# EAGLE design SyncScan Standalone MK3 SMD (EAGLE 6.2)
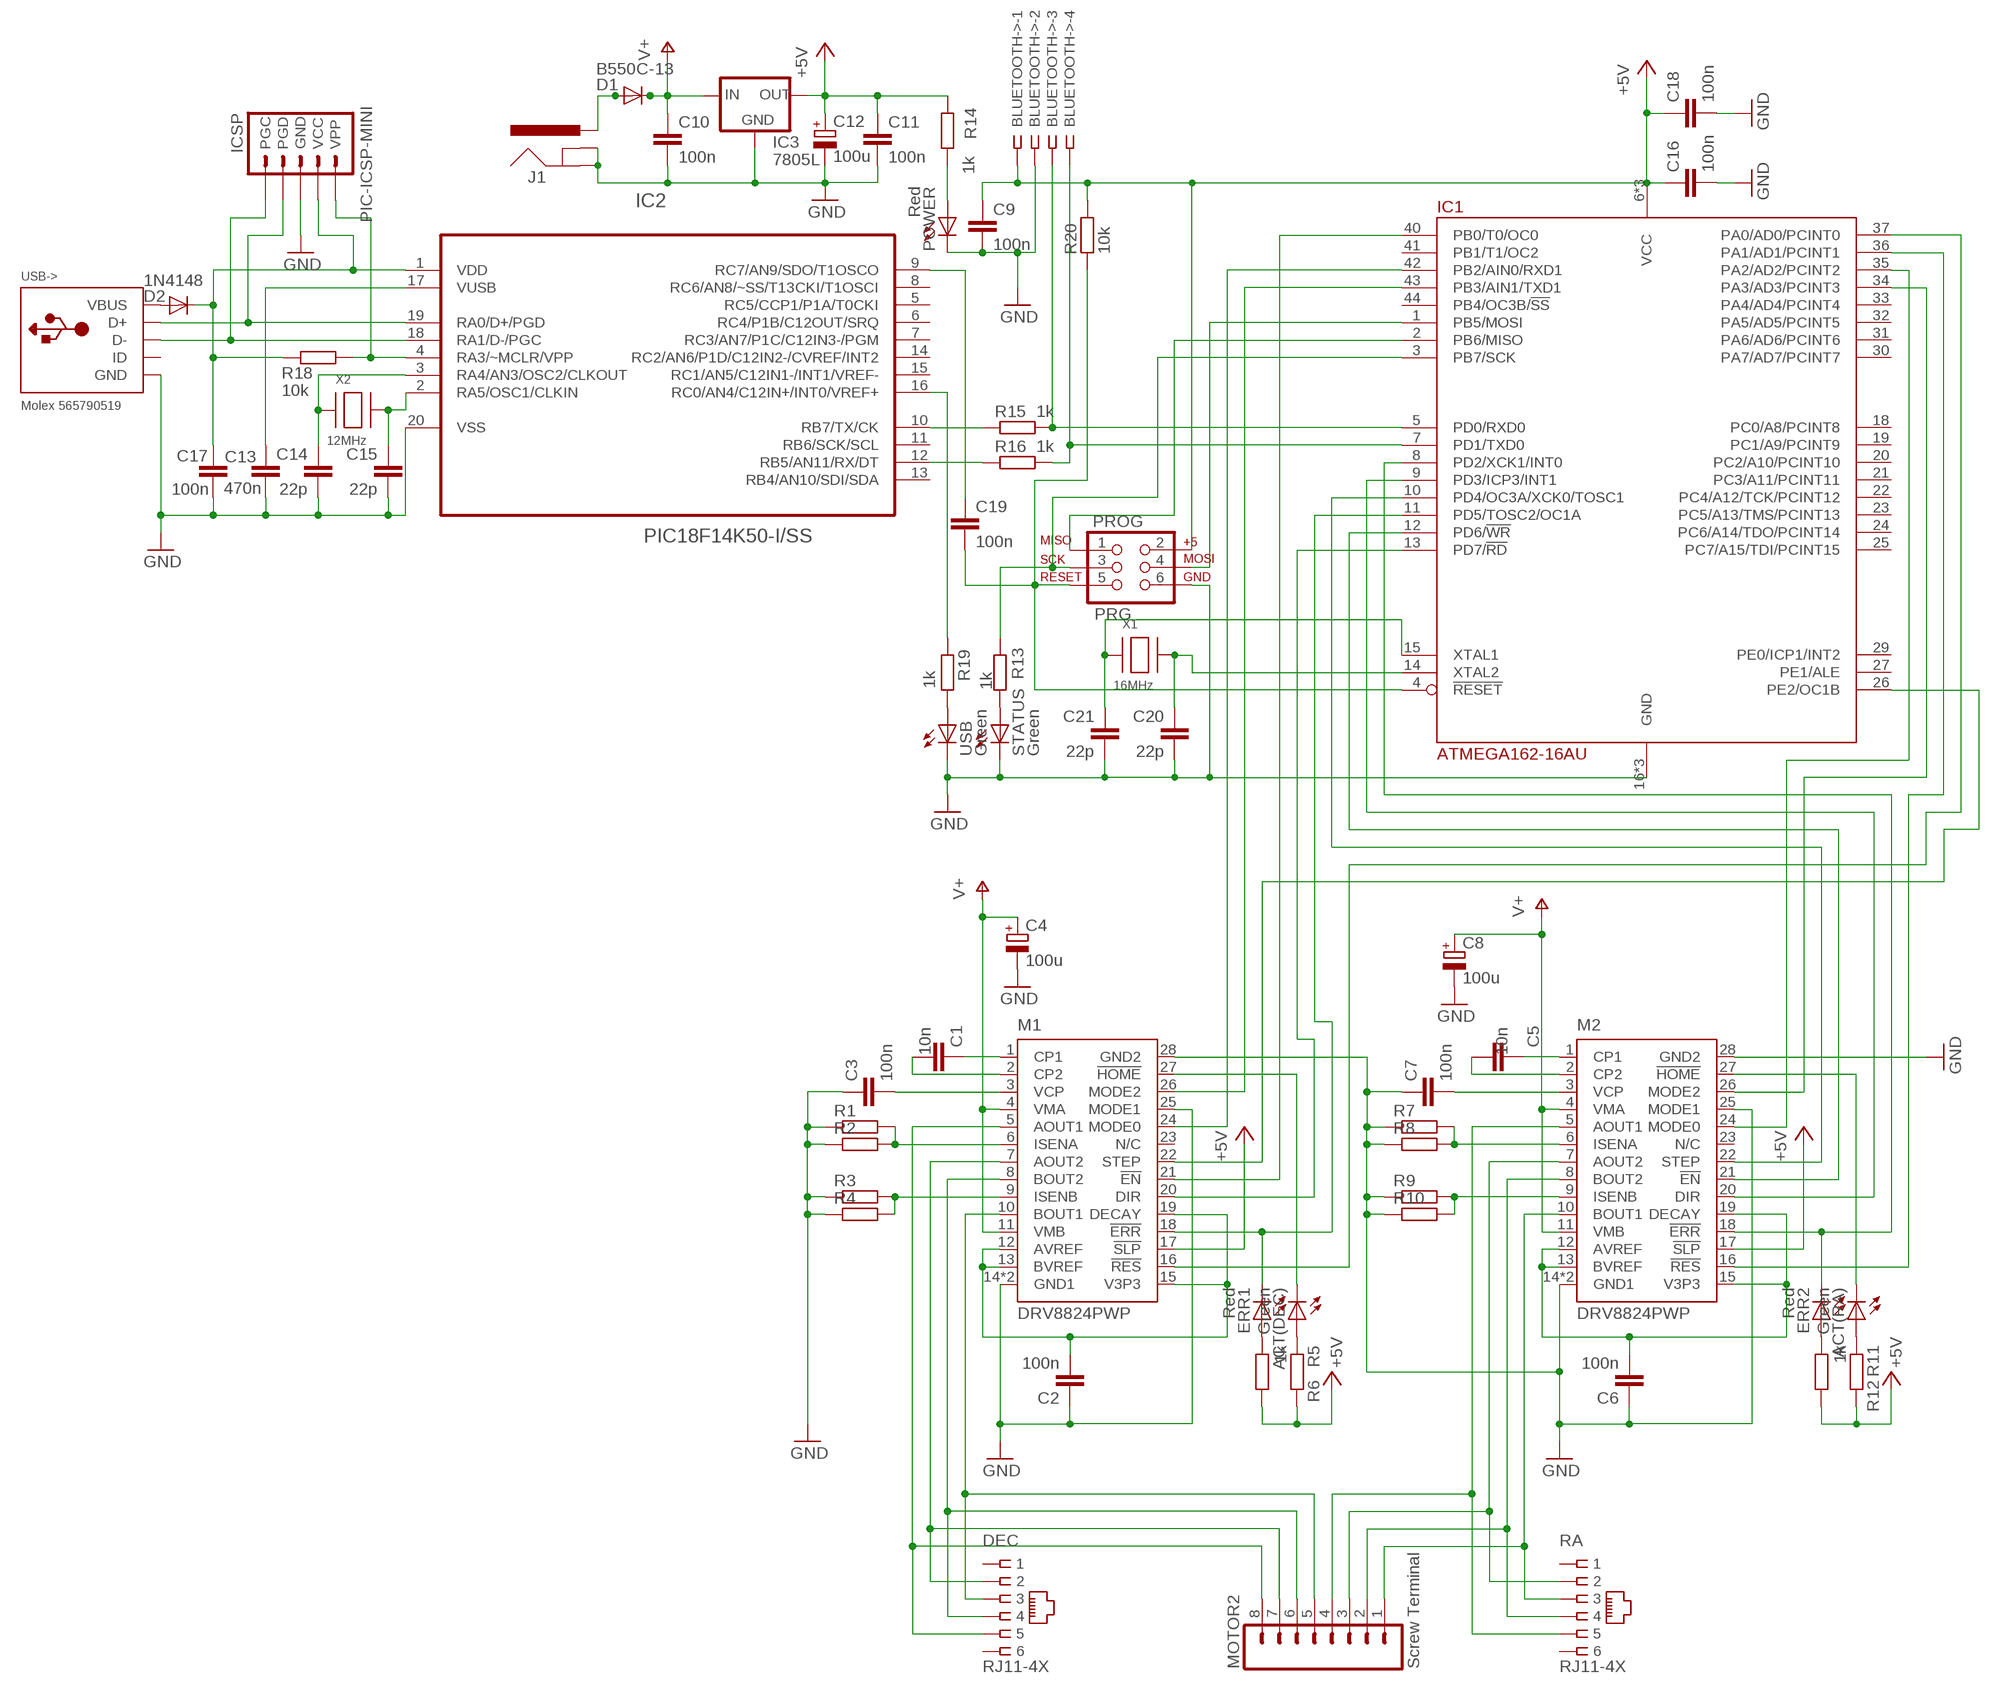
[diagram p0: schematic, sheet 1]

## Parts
ACT(DEC)  Green  LEDSMT1206  [1206]
ACT(RA)  Green  LEDSMT1206  [1206]
BLUETOOTH->  http://www.ebay.co.uk/itm/250991624201  SSW-104-02-S-S-RA  [SSW-104-02-S-S-RA]
C1  10n  C-EUC0603K  [C0603K]
C2  100n  C-EUC0603K  [C0603K]
C3  100n  C-EUC0603K  [C0603K]
C4  100u  CPOL-EUE2.5-6  [E2,5-6]
C5  10n  C-EUC0603K  [C0603K]
C6  100n  C-EUC0603K  [C0603K]
C7  100n  C-EUC0603K  [C0603K]
C8  100u  CPOL-EUE2.5-6  [E2,5-6]
C9  100n  C-EUC0603K  [C0603K]
C10  100n  C-EUC0603K  [C0603K]
C11  100n  C-EUC0603K  [C0603K]
C12  100u  CPOL-EUE2.5-6  [E2,5-6]
C13  470n  C-EUC0603K  [C0603K]
C14  22p  C-EUC0603K  [C0603K]
C15  22p  C-EUC0603K  [C0603K]
C16  100n  C-EUC0603K  [C0603K]
C17  100n  C-EUC0603K  [C0603K]
C18  100n  C-EUC0603K  [C0603K]
C19  100n  C-EUC0603K  [C0603K]
C20  22p  C-EUC0603K  [C0603K]
C21  22p  C-EUC0603K  [C0603K]
D1  B550C-13  DIODE-SMC  [SMC]
D2  1N4148  DIODESOD  [SOD-323]
DEC  RJ11-4X  [RJ11-NO_SHIELD]
ERR1  Red  LEDSMT1206  [1206]
ERR2  Red  LEDSMT1206  [1206]
IC1  ATMEGA162-16AU  [TQFP44]
IC2  PIC18F14K50-I/SS  [SSOP20]
IC3  7805L  78LXXSOT-23  [SOT23]
ICSP  PIC-ICSP-MINI  [PIC-ICSP-MINI]
J1  POWER_JACKSMD  [POWER_JACK_SMD]
M1  DRV8824PWP  [HTSSOP28PWP]
M2  DRV8824PWP  [HTSSOP28PWP]
MOTOR2  Screw Terminal  M083.5MM-8  [SCREWTERMINAL-3.5MM-8]
POWER  Red  LEDSMT1206  [1206]
PROG  PRG  AVR_SPI_PRG_6PTH  [2X3]
R1  1.5R  R-EU_R2512  [R2512]
R2  1.5R  R-EU_R2512  [R2512]
R3  1.5R  R-EU_R2512  [R2512]
R4  1.5R  R-EU_R2512  [R2512]
R5  1k  R-EU_R0603  [R0603]
R6  1k  R-EU_R0603  [R0603]
R7  1.5R  R-EU_R2512  [R2512]
R8  1.5R  R-EU_R2512  [R2512]
R9  1.5R  R-EU_R2512  [R2512]
R10  1.5R  R-EU_R2512  [R2512]
R11  1k  R-EU_R0603  [R0603]
R12  1k  R-EU_R0603  [R0603]
R13  1k  R-EU_R0603  [R0603]
R14  1k  R-EU_R0603  [R0603]
R15  1k  R-EU_R0603  [R0603]
R16  1k  R-EU_R0603  [R0603]
R18  10k  R-EU_R0603  [R0603]
R19  1k  R-EU_R0603  [R0603]
R20  10k  R-EU_R0603  [R0603]
RA  RJ11-4X  [RJ11-NO_SHIELD]
STATUS  Green  LEDSMT1206  [1206]
USB  Green  LEDSMT1206  [1206]
USB->  Molex 565790519  USBMOLEX  [USB-MINIB-THM-MOLEX]
X1  16MHz  XTALNX5032  [NX5032]
X2  12MHz  XTALNX5032  [NX5032]

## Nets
3.3V-1: C2.2 M1.12(AVREF) M1.13(BVREF) M1.15(V3P3) M1.19(DECAY)
3.3V-2: C6.2 M2.12(AVREF) M2.13(BVREF) M2.15(V3P3) M2.19(DECAY)
!EN-1: IC1.40(PB0/T0/OC0) M1.21(!EN)
!EN-2: IC1.12(PD6/!WR) M2.21(!EN)
!ERR-1: ERR1.C IC1.11(PD5/TOSC2/OC1A) M1.18(!ERR)
!ERR-2: ERR2.C IC1.8(PD2/XCK1/INT0) M2.18(!ERR)
!HOME-1: ACT(DEC).C M1.27(!HOME)
!HOME-2: ACT(RA).C M2.27(!HOME)
!RST-1: IC1.37(PA0/AD0/PCINT0) M1.16(!RES)
!RST-2: IC1.36(PA1/AD1/PCINT1) M2.16(!RES)
+5V: BLUETOOTH->.1 C9.1 C11.1 C12.+ C16.1 C18.1 IC1.6(VCC) IC1.17(VCC) IC1.38(VCC) IC3.1(OUT) M1.17(!SLP) M2.17(!SLP) PROG.2 R5.2 R6.2 R11.2 R12.2 R14.1 R20.2
A1-1: DEC.5 M1.5(AOUT1) MOTOR2.8
A1-2: M2.5(AOUT1) MOTOR2.4 RA.5
A2-1: DEC.2 M1.7(AOUT2) MOTOR2.7
A2-2: M2.7(AOUT2) MOTOR2.3 RA.2
AVROSC1: C21.1 IC1.15(XTAL1) X1.P$1
AVROSC2: C20.1 IC1.14(XTAL2) X1.P$2
B1-1: DEC.3 M1.10(BOUT1) MOTOR2.5
B1-2: M2.10(BOUT1) MOTOR2.1 RA.3
B2-1: DEC.4 M1.8(BOUT2) MOTOR2.6
B2-2: M2.8(BOUT2) MOTOR2.2 RA.4
CP1-1: C1.1 M1.1(CP1)
CP1-2: C5.1 M2.1(CP1)
CP2-1: C1.2 M1.2(CP2)
CP2-2: C5.2 M2.2(CP2)
D+: IC2.19(RA0/D+/PGD) ICSP.4(PGD) USB->.D+
D-: IC2.18(RA1/D-/PGC) ICSP.5(PGC) USB->.D-
DIR-1: IC1.13(PD7/!RD) M1.20(DIR)
DIR-2: IC1.9(PD3/ICP3/INT1) M2.20(DIR)
GND: BLUETOOTH->.2 C2.1 C3.1 C4.- C6.1 C7.1 C8.- C9.2 C10.2 C11.2 C12.- C13.1 C14.2 C15.2 C16.2 C17.2 C18.2 C20.2 C21.2 IC1.16(GND) IC1.28(GND) IC1.39(GND) IC2.20(VSS) IC3.3(GND) ICSP.3(GND) J1.GND(GNDBREAK) J1.P$4(GND) M1.14(GND1) M1.25(MODE1) M1.28(GND2) M1.EXP(GND1) M2.14(GND1) M2.25(MODE1) M2.28(GND2) M2.EXP(GND1) POWER.C PROG.6 R1.1 R2.1 R3.1 R4.1 R7.1 R8.1 R9.1 R10.1 STATUS.C USB->.GND USB.C
ISENA-1: M1.6(ISENA) R1.2 R2.2
ISENA-2: M2.6(ISENA) R7.2 R8.2
ISENB-1: M1.9(ISENB) R3.2 R4.2
ISENB-2: M2.9(ISENB) R9.2 R10.2
LED1: ERR1.A R6.1
LED2: ACT(DEC).A R5.1
LED3: ERR2.A R12.1
LED4: ACT(RA).A R11.1
M0-1: IC1.42(PB2/AIN0/RXD1) M1.24(MODE0)
M0-2: IC1.35(PA2/AD2/PCINT2) M2.24(MODE0)
M2-1: IC1.43(PB3/AIN1/TXD1) M1.26(MODE2)
M2-2: IC1.34(PA3/AD3/PCINT3) M2.26(MODE2)
MCLR: IC2.4(RA3/~MCLR/VPP) ICSP.1(VPP) R18.1
MISO: IC1.2(PB6/MISO) PROG.1
MOSI: IC1.1(PB5/MOSI) PROG.4
N$1: C3.2 M1.3(VCP)
N$2: C19.1 IC2.9(RC7/AN9/SDO/T1OSCO)
PWRLED: POWER.A R14.2
RESET: C19.2 IC1.4(!RESET) PROG.5 R20.1
RX(BTH): BLUETOOTH->.4 IC1.7(PD1/TXD0) R16.1
RX(USB): IC2.12(RB5/AN11/RX/DT) R16.2
SCLK: IC1.3(PB7/SCK) PROG.3 R13.1
STATLED: R13.2 STATUS.A
STEP-1: IC1.26(PE2/OC1B) M1.22(STEP)
STEP-2: IC1.10(PD4/OC3A/XCK0/TOSC1) M2.22(STEP)
TX(BTH): BLUETOOTH->.3 IC1.5(PD0/RXD0) R15.1
TX(USB): IC2.10(RB7/TX/CK) R15.2
USBLED: R19.1 USB.A
USBOSC1: C15.1 IC2.2(RA5/OSC1/CLKIN) X2.P$2
USBOSC2: C14.1 IC2.3(RA4/AN3/OSC2/CLKOUT) X2.P$1
USBSTAT: IC2.16(RC0/AN4/C12IN+/INT0/VREF+) R19.2
V+: C4.+ C8.+ C10.1 D1.C IC3.2(IN) M1.4(VMA) M1.11(VMB) M2.4(VMA) M2.11(VMB)
VBUS: D2.2(A) USB->.VBUS
VCP-2: C7.2 M2.3(VCP)
VIN: D1.A J1.VIN0(PWR) J1.VIN1(PWR)
VPIC: C17.1 D2.1(C) IC2.1(VDD) ICSP.2(VCC) R18.2
VUSB: C13.2 IC2.17(VUSB)
Unconnected: DEC.1 DEC.6 IC1.18(PC0/A8/PCINT8) IC1.19(PC1/A9/PCINT9) IC1.20(PC2/A10/PCINT10) IC1.21(PC3/A11/PCINT11) IC1.22(PC4/A12/TCK/PCINT12) IC1.23(PC5/A13/TMS/PCINT13) IC1.24(PC6/A14/TDO/PCINT14) IC1.25(PC7/A15/TDI/PCINT15) IC1.27(PE1/ALE) IC1.29(PE0/ICP1/INT2) IC1.30(PA7/AD7/PCINT7) IC1.31(PA6/AD6/PCINT6) IC1.32(PA5/AD5/PCINT5) IC1.33(PA4/AD4/PCINT4) IC1.41(PB1/T1/OC2) IC1.44(PB4/OC3B/!SS) IC2.5(RC5/CCP1/P1A/T0CKI) IC2.6(RC4/P1B/C12OUT/SRQ) IC2.7(RC3/AN7/P1C/C12IN3-/PGM) IC2.8(RC6/AN8/~SS/T13CKI/T1OSCI) IC2.11(RB6/SCK/SCL) IC2.13(RB4/AN10/SDI/SDA) IC2.14(RC2/AN6/P1D/C12IN2-/CVREF/INT2) IC2.15(RC1/AN5/C12IN1-/INT1/VREF-) M1.23(N/C) M2.23(N/C) RA.1 RA.6 USB->.ID

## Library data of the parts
ACT(DEC) ACT(RA) STATUS USB = led:LED: LED; MF: KINGBRIGHT; MPN: L-424GDT; OC_FARNELL: 1142496
BLUETOOTH-> = con-samtec:SSW-104-02-S-S: THROUGH-HOLE .025" SQ POST SOCKET Source: Samtec SSW.pdf; OC_FARNELL: unknown; OC_NEWARK: 11P9385
C1 C5 = resistor:C-EU: CAPACITOR, European symbol; MF: KEMET; MPN: C0603C103K1RACTU; OC_FARNELL: 1865545
C2 C3 C6 C7 C9-C11 C16-C19 = resistor:C-EU: CAPACITOR, European symbol; MF: KEMET; MPN: C0603C104K4RACTU; OC_FARNELL: 1414610
C4 C8 C12 = resistor:CPOL-EU: POLARIZED CAPACITOR, European symbol; MF: MULTICOMP; MPN: MCGPR25V107M6.3X11; OC_FARNELL: 9451188
C13 = rcl:C-EU: CAPACITOR, European symbol; MF: AVX; MPN: 0603ZD474KAT2A; OC_FARNELL: 1833805
C14 C15 C20 C21 = rcl:C-EU: CAPACITOR, European symbol; MF: MULTICOMP; MPN: U0603C220JCT; OC_FARNELL: 9406107
D1 = diode:DIODE-: DIODE; MF: DIODES INC.; MPN: B550C-13-F; OC_FARNELL: 1858608
D2 = SparkFun:DIODE: Diode; MF: MULTICOMP; MPN: 1N4148.; OC_FARNELL: 9565124
DEC RA = con-tycoelectronics:RJ11: CORCOM Modular RJ Jacks No Shield Source: www.tycoelectronics.com .. ENG_DS_1654001_1099_RJ_L_0507.pdf; MF: MH CONNECTORS; MPN: MHRJJ64NFRA; OC_FARNELL: 3938347; OC_NEWARK: 19R7022
ERR1 ERR2 POWER = led:LED: LED; MF: KINGBRIGHT; MPN: L-424HDT; OC_FARNELL: 1142499
IC1 = atmel:ATMEGA162: 8-bit RISC MICROCONTROLLER 16K Bytes internal flash program memory 1K Bytes internal SRAM Upto 64K Bytes optional external memory space 512 Bytes EEPROM Two 8-bit timers Two 16-bit timers Dual programmable serial USARTs Master/Slave serial SPI interface Source: ATMEGA162_DIP40.lbr; MF: ATMEL; MPN: ATMEGA162-16AU; OC_FARNELL: 9171150
IC2 = microchip:PIC18F14K50: USB Flash Microcontrollers; MF: MICROCHIP; MPN: PIC18F14K50-I/SS; OC_FARNELL: 1648504
IC3 = v-reg:78LXX: VOLTAGE REGULATOR; MF: TAIWAN SEMICONDUCTOR; MPN: TS78L05CX RF; OC_FARNELL: 1476698
ICSP = SparkFun:PIC-ICSP-MINI: PIC-ICSP-Mini Miniature 5-pin connection for temporary programming of PICs. Use this device in your design to save space. Program the PIC with this adapter Spark Fun Electronics SKU : BOB-00194; OC_FARNELL: unknown
J1 = SparkFun:POWER_JACK: Power Jack This is the standard 5.5mm barrel jack for power. The PTH is the most common, proven, reliable, footprint. All others are experimental. The Slot footprint only works if the mill layer is transmitted to the PCB fab house so be warned. Spark Fun Electronics SKU : PRT-00119. Mating wall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; MF: MULTICOMP; MPN: MJ-179SMT; OC_FARNELL: 1737262
M1 M2 = texas:DRV8824; MF: TEXAS INSTRUMENTS; MPN: DRV8824PWP; OC_FARNELL: 1815786
MOTOR2 = SparkFun:M08: Header 8 Standard 8-pin 0.1" header. Use with straight break away headers (SKU : PRT-00116), right angle break away headers (PRT-00553), swiss pins (PRT-00743), machine pins (PRT-00117), and female headers (PRT-00115).; MF: LUMBERG; MPN: KRMC 08; OC_FARNELL: 1217307
PROG = SparkFun:AVR_SPI_PRG_6: AVR ISP 6 Pin This is the reduced ISP connector for AVR programming. Common on Arduino. This footprint will take up less PCB space and can be used with a 10-pin to 6-pin adapter such as SKU: BOB-08508; MF: TE CONNECTIVITY / AMP; MPN: 826632-3; OC_FARNELL: 3418492
R1-R4 R7-R10 = resistor:R-EU_: RESISTOR, European symbol; MF: YAGEO (PHYCOMP); MPN: RC2512FK-7W1R5L; OC_FARNELL: 1840520
R5 R6 R11 R12 = resistor:R-EU_: RESISTOR, European symbol; MF: VISHAY DRALORIC; MPN: CRCW06031K00FKEA; OC_FARNELL: 1469740
R13 R14 R19 = rcl:R-EU_: RESISTOR, European symbol; MF: VISHAY DRALORIC; MPN: CRCW06031K00FKEA; OC_FARNELL: 1469740
R15 R16 = SmartPrj:R-EU_: RESISTOR, European symbol; MF: VISHAY DRALORIC; MPN: CRCW06031K00FKEA; OC_FARNELL: 1469740
R18 R20 = rcl:R-EU_: RESISTOR, European symbol; MF: VISHAY DRALORIC; MPN: CRCW060310K0FKEA; OC_FARNELL: 1469748
USB-> = adafruit:USB: USB Connectors USBMINIB - Surface Mount Female Mini-B USB Connector 4UConnector: 06564 By microbuilder.eu Thru-hole RA Female Mini-B USB Connector 4UConnector: 18732 By ladyada.net; MF: MOLEX; MPN: 565790519; OC_FARNELL: 1125347
X1 = adafruit:XTAL: Low cost SMT crystals, no capacitors included; MF: TXC; MPN: 7A-16.000MAAJ-T; OC_FARNELL: 1841946
X2 = adafruit:XTAL: Low cost SMT crystals, no capacitors included; MF: TXC; MPN: 7A-12.000MAAJ-T; OC_FARNELL: 1841940

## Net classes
1 power: width 0.61 mm, drill 0.711 mm, clearance 0.203 mm
2 gnd: width 0.305 mm, drill 0.711 mm, clearance 0.203 mm
3 usbvcc: width 0.508 mm, drill 0.711 mm, clearance 0.203 mm

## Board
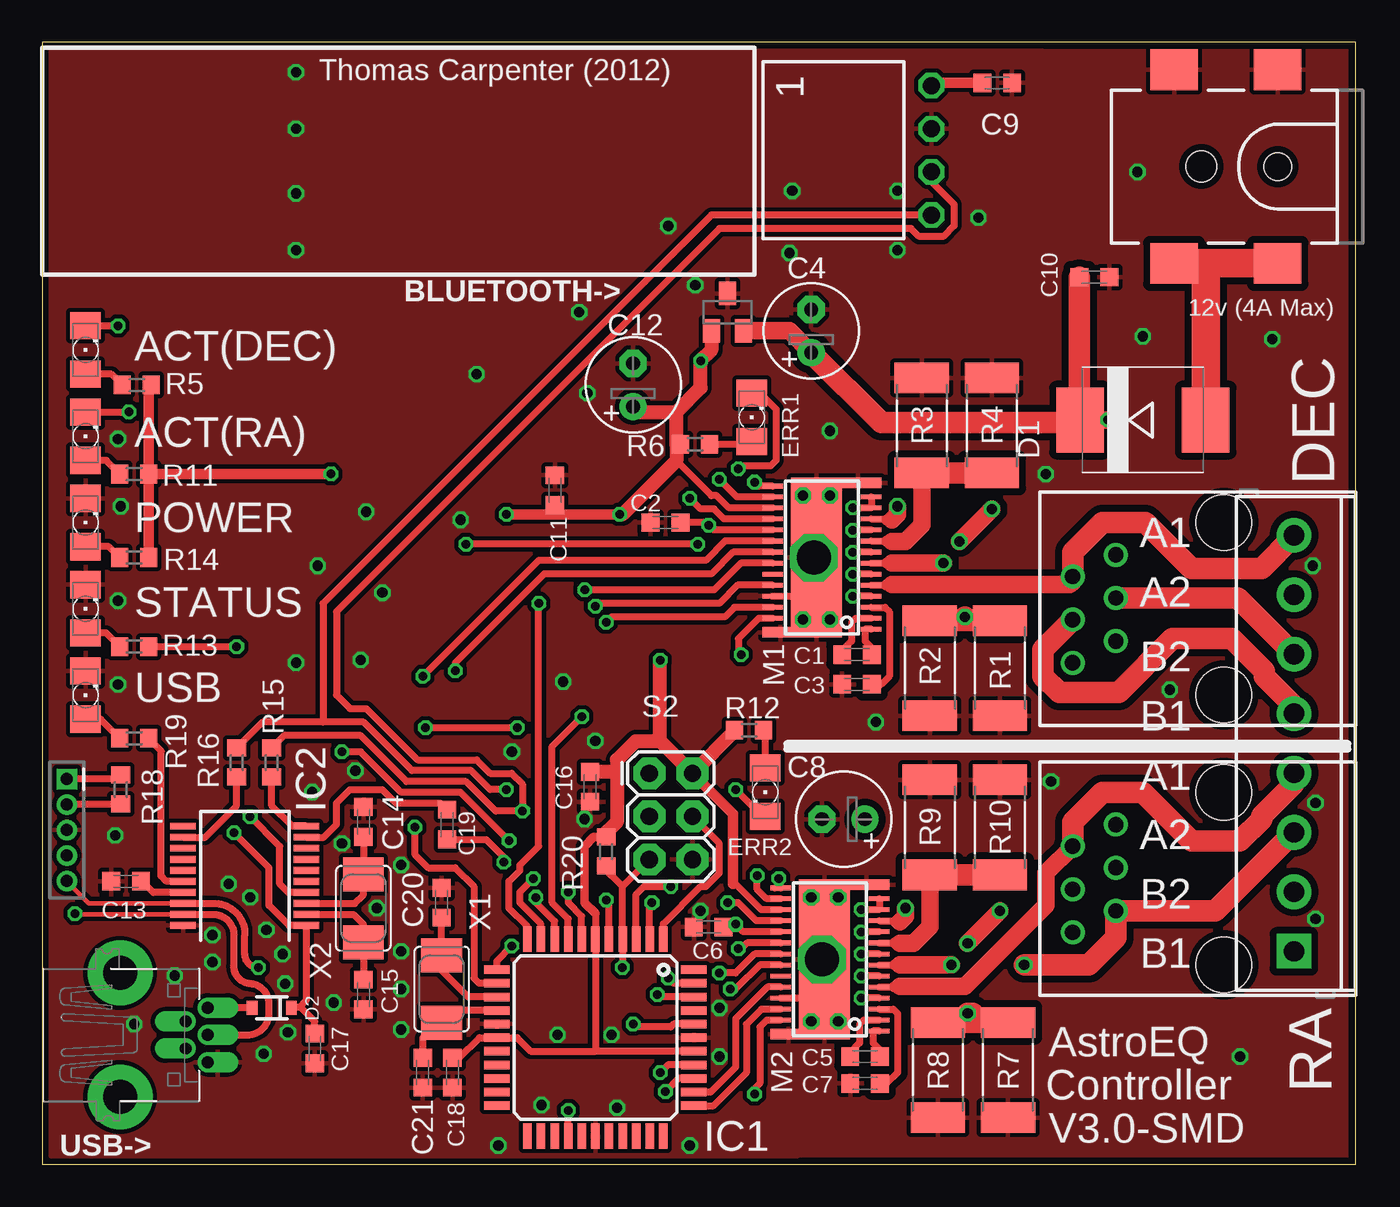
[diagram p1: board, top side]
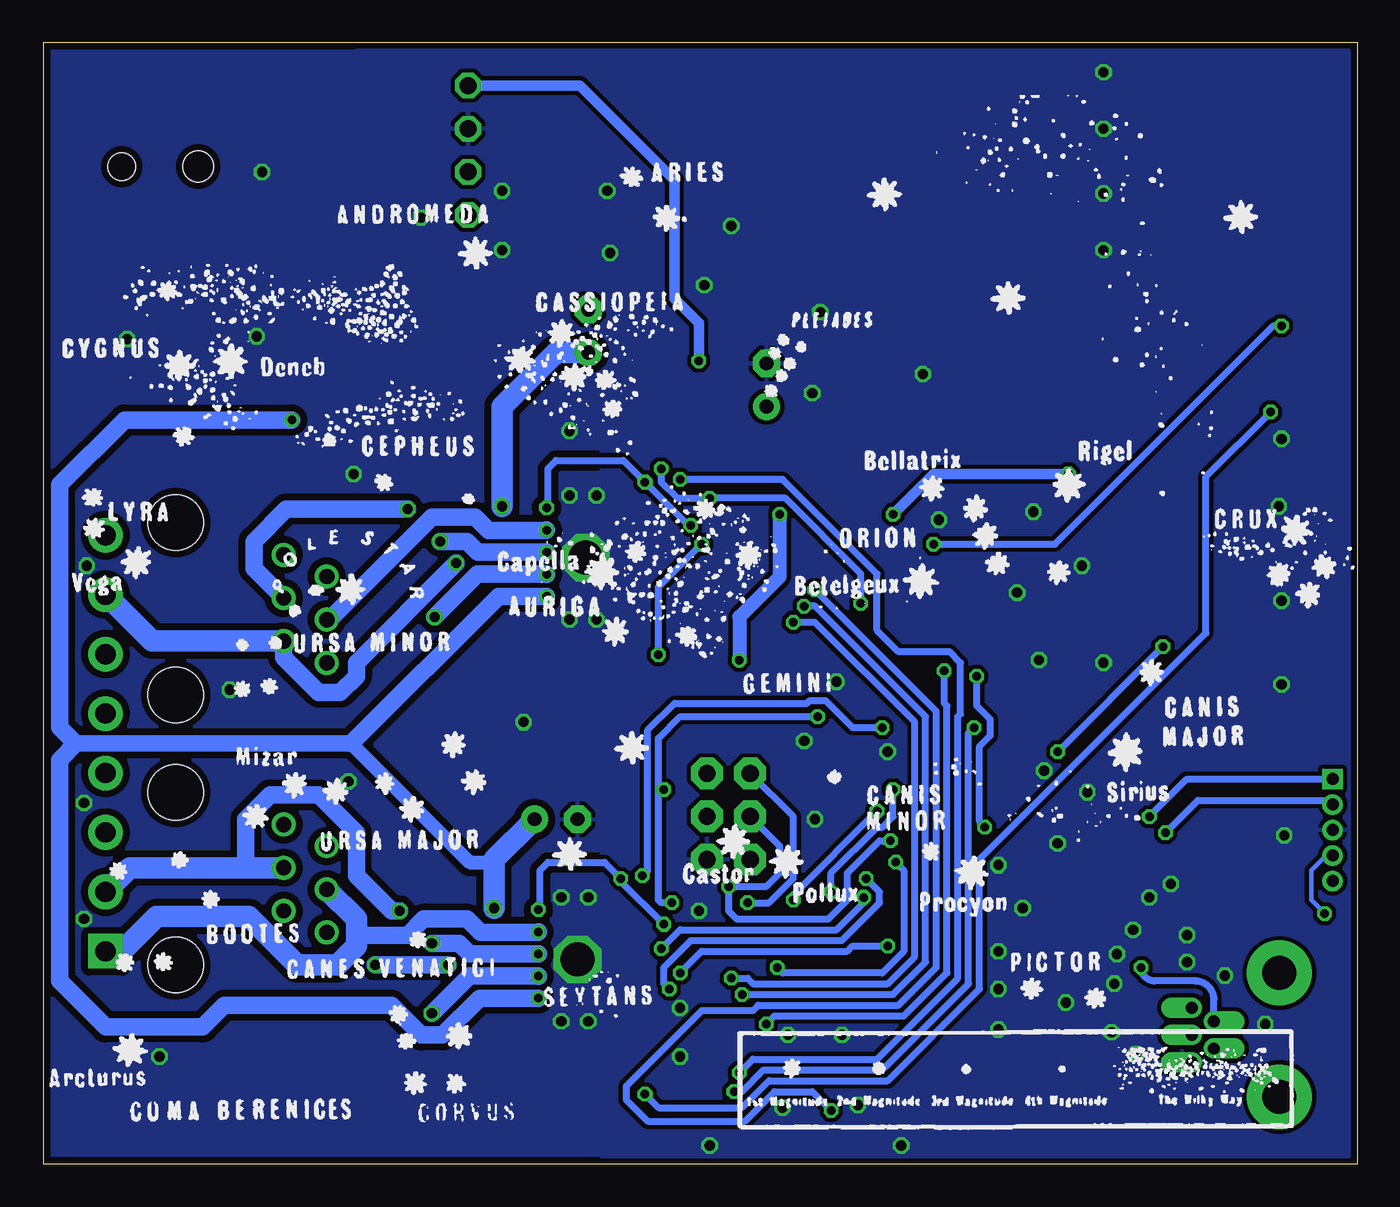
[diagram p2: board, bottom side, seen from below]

Size 77.31 x 66.04 mm. Coordinates in mm from the lower left corner, seen from the top.
Outline: 0,66.04 0,0 77.31,0 77.31,66.04 0,66.04
Copper layers (1*16): Top 0.035mm / dielectric 1.5mm / Bottom 0.035mm
Design rules: minimum track width 0.2mm, minimum drill 0.5mm, track to track 0.2mm, track to pad 0.2mm, pad to pad 0.2mm, via to via 0.2mm, smd to smd 0mil, copper to edge 10mil, drill to drill 0.2mm, minimum pad ring 10mil, minimum via ring 7mil, stop-mask expansion 0.125mm, vias tented up to drill 0mil, thermal gap 10mil

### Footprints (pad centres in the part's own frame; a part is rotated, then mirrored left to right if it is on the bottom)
1206 = smd 1.6 x 1.803: A -1.422,0; C 1.422,0
SSW-104-02-S-S-RA = drill 1 pad 1.5 octagon: 1 -3.81,1.524; 2 -1.27,1.524; 3 1.27,1.524; 4 3.81,1.524
C0603K = smd 1.05 x 1.08: 1 -0.875,0; 2 0.875,0
E2,5-6 = drill 0.813 pad 1.6: + -1.27,0 | drill 0.813 pad 1.6 octagon: - 1.27,0
SMC = smd 2.8 x 3.8: A 3.7,0; C -3.7,0
SOD-323 = smd 0.63 x 0.83: 1 -1.15,0; 2 1.15,0
RJ11-NO_SHIELD = drill 0.9 pad 1.4: 1 -3.175,8.89; 2 -1.905,6.35; 3 -0.635,8.89; 4 0.635,6.35; 5 1.905,8.89; 6 3.175,6.35 | hole 3.251: -5.08,0; 5.08,0
TQFP44 = smd 1.5 x 0.5: 1 -5.8,4; 2 -5.8,3.2; 3 -5.8,2.4; 4 -5.8,1.6; 5 -5.8,0.8; 6 -5.8,0; 7 -5.8,-0.8; 8 -5.8,-1.6; 9 -5.8,-2.4; 10 -5.8,-3.2; 11 -5.8,-4; 23 5.8,-4; 24 5.8,-3.2; 25 5.8,-2.4; 26 5.8,-1.6; 27 5.8,-0.8; 28 5.8,0; 29 5.8,0.8; 30 5.8,1.6; 31 5.8,2.4; 32 5.8,3.2; 33 5.8,4 | smd 0.5 x 1.5: 12 -4,-5.8; 13 -3.2,-5.8; 14 -2.4,-5.8; 15 -1.6,-5.8; 16 -0.8,-5.8; 17 0,-5.8; 18 0.8,-5.8; 19 1.6,-5.8; 20 2.4,-5.8; 21 3.2,-5.8; 22 4,-5.8; 34 4,5.8; 35 3.2,5.8; 36 2.4,5.8; 37 1.6,5.8; 38 0.8,5.8; 39 0,5.8; 40 -0.8,5.8; 41 -1.6,5.8; 42 -2.4,5.8; 43 -3.2,5.8; 44 -4,5.8
SSOP20 = smd 0.4 x 1.5: 1 -2.925,-3.625; 2 -2.275,-3.625; 3 -1.625,-3.625; 4 -0.975,-3.625; 5 -0.325,-3.625; 6 0.325,-3.625; 7 0.975,-3.625; 8 1.625,-3.625; 9 2.275,-3.625; 10 2.925,-3.625; 11 2.925,3.625; 12 2.275,3.625; 13 1.625,3.625; 14 0.975,3.625; 15 0.325,3.625; 16 -0.325,3.625; 17 -0.975,3.625; 18 -1.625,3.625; 19 -2.275,3.625; 20 -2.925,3.625
SOT23 = smd 1 x 1.4: 1 -0.95,-1.1; 2 0.95,-1.1; 3 0,1.1
PIC-ICSP-MINI = drill 0.7 square: 1 -3,0 | drill 0.7: 2 -1.5,0; 3 0,0; 4 1.5,0; 5 3,0
POWER_JACK_SMD = smd 2.8 x 2.4: GND 0,-5.7; P$4 6.1,-5.7; VIN0 0,5.7; VIN1 6.1,5.7 | hole 1.6: 0,0 | hole 1.8: 4.5,0
HTSSOP28PWP = smd 0.27 x 1.2: 1 -4.21,-2.9; 2 -3.575,-2.9; 3 -2.925,-2.9; 4 -2.275,-2.9; 5 -1.625,-2.9; 6 -0.975,-2.9; 7 -0.325,-2.9; 8 0.325,-2.9; 9 0.975,-2.9; 10 1.625,-2.9; 11 2.275,-2.9; 12 2.925,-2.9; 13 3.575,-2.9; 15 4.21,2.9; 16 3.575,2.9; 17 2.925,2.9; 18 2.275,2.9; 19 1.625,2.9; 20 0.975,2.9; 21 0.325,2.9; 22 -0.325,2.9; 23 -0.975,2.9; 24 -1.625,2.9; 25 -2.275,2.9; 26 -2.925,2.9; 27 -3.575,2.9 | smd 0.61 x 2.735: 14 4.395,-2.132 | smd 0.61 x 2.1: 28 -4.395,2.45 | smd 9.4 x 3: EXP 0,0.318
SCREWTERMINAL-3.5MM-8 = drill 1.2 pad 2.032 square: 1 0,0 | drill 1.2 pad 2.032: 2 3.5,0; 3 7,0; 4 10.5,0; 5 14,0; 6 17.5,0; 7 21,0; 8 24.5,0
2X3 = drill 1.016 pad 1.88 octagon: 1 0,0; 2 0,2.54; 3 2.54,0; 4 2.54,2.54; 5 5.08,0; 6 5.08,2.54
R2512 = smd 1.8 x 3.2: 1 -2.8,0; 2 2.8,0
R0603 = smd 1 x 1.1: 1 -0.85,0; 2 0.85,0
USB-MINIB-THM-MOLEX = drill 0.7 offset: D+ 0,9.72; D- -0.8,8.42; GND 1.6,9.72; ID 0.8,8.42; VBUS -1.6,9.72 | drill 2 pad 3.81: GND1 -3.65,4.57; GND4 3.65,4.57
NX5032 = smd 2 x 2.4: P$1 2,0; P$2 -2,0

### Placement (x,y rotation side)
ACT(DEC)  2.54,47.94 90 top
ACT(RA)  2.54,42.86 90 top
BLUETOOTH->  50.8,59.69 270 top
C1  47.94,30 180 top
C2  36.67,37.78 0 top
C3  47.94,28.26 0 top
C4  45.24,49.05 90 top
C5  48.42,6.35 180 top
C6  39.21,13.97 0 top
C7  48.42,4.76 0 top
C8  47.15,20.32 180 top
C9  56.2,63.66 0 top
C10  61.91,52.23 0 top
C11  30.16,39.69 90 top
C12  34.77,45.88 90 top
C13  4.92,16.67 0 top
C14  18.89,20.16 90 top
C15  18.89,10 270 top
C16  32.23,22.23 270 top
C17  16.03,6.83 270 top
C18  24.13,5.4 270 top
C19  23.81,20 270 top
C20  23.5,15.4 90 top
C21  22.38,5.4 270 top
D1  64.77,43.81 0 top
D2  13.49,9.21 180 top
DEC  69.53,32.7 90 top
ERR1  41.75,43.97 90 top
ERR2  42.55,21.91 270 top
IC1  32.54,7.46 270 top
IC2  11.91,16.99 90 top
IC3  40.32,50.16 0 top
ICSP  1.43,19.68 270 top
J1  72.71,58.74 180 top
M1  45.88,35.72 90 top
M2  46.35,12.06 90 top
MOTOR2  73.66,12.54 90 top
POWER  2.54,37.78 90 top
PROG  35.72,23.02 270 top
R1  56.36,29.21 90 top
R2  52.23,29.21 90 top
R3  51.75,43.5 270 top
R4  55.88,43.5 270 top
R5  5.56,45.88 0 top
R6  38.42,42.39 180 top
R7  56.83,5.56 90 top
R8  52.7,5.56 90 top
R9  52.23,19.84 270 top
R10  56.36,19.84 270 top
R11  5.4,40.64 0 top
R12  41.59,25.56 180 top
R13  5.4,30.48 180 top
R14  5.4,35.72 180 top
R15  13.49,23.65 270 top
R16  11.43,23.65 270 top
R18  4.6,22.07 270 top
R19  5.4,25.08 0 top
R20  33.18,18.41 90 top
RA  69.53,16.83 90 top
STATUS  2.54,32.7 90 top
USB  2.54,27.62 90 top
USB->  0,7.62 270 top
X1  23.5,10.32 270 top
X2  18.89,15.08 90 top

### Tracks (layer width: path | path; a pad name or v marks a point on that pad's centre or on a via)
3.3V-1  (via drill 0.5)
  Top 0.406: v47.7,38.66 47.72,38.64 M1.12 M1.13 | M1.15 42.15,39.93 v41.91,40.16 | M1.19 39.49,37.34 v39.21,37.62 39.05,37.78 C2.2
  Bottom 0.406: v47.7,38.66 47.62,38.73 47.62,40.96 47.15,41.43 43.18,41.43 v41.91,40.16 39.37,37.62 v39.21,37.62
3.3V-2  (via drill 0.5)
  Top 0.406: v48.18,15 48.19,14.99 M2.12 M2.13 | 43.1,16.27 M2.15 43.45,16.39 43.34,16.51 v43.34,16.83 | M2.19 41.24,13.69 v40.8,14.13 40.64,13.97 C6.2
  Bottom 0.406: v48.18,15 48.1,15.08 48.1,17.3 47.62,17.78 44.29,17.78 v43.34,16.83 43.34,16.67 v40.8,14.13
!EN-1  (via drill 0.5)
  Top 0.406: M1.21 40.65,36.04 39.37,34.77 29.53,34.77 24.29,29.53 v24.29,29.05 | IC1.40 37.15,8.26 36.99,8.1 34.92,8.1 v34.77,8.26 v34.76,8.26
  Bottom 0.406: v34.77,8.26 34.29,8.73 26.67,8.73 24.13,11.27 24.13,26.99 24.29,27.15 v24.29,29.05
!EN-2  (via drill 0.5)
  Top 0.406: M2.21 41.92,12.39 40.8,11.27 v39.85,11.27 | IC1.12 26.74,11.98 v27.62,12.86
  Bottom 0.406: v39.85,11.27 38.58,12.54 30,12.54 29.69,12.86 v27.62,12.86
!ERR-1  (via drill 0.5)
  Top 0.406: M1.18 40.11,37.99 39.53,38.58 38.73,38.58 v38.1,39.21 | IC1.11 28.54,14 27.46,15.08 27.46,16.67 28.1,17.3 28.1,17.62 29.21,18.73 v29.21,33.02 | ERR1.C 42.23,45.4 43.18,44.45 43.18,41.43 42.86,41.12 41.12,41.12 v40.96,40.96
  Bottom 0.406: v29.21,33.02 29.21,34.77 33.66,39.21 v38.1,39.21 40.01,39.21 40.96,40.16 v40.96,40.96
!ERR-2  (via drill 0.5)
  Top 0.406: M2.18 42.02,14.34 40.96,15.4 v40.32,15.4 | IC1.8 30.94,14.46 30,15.4 30,24.61 v31.75,26.35 | ERR2.C 42.06,20.48 42.07,20.48 42.07,20.8 v40.8,22.07
  Bottom 0.406: v40.32,15.4 40.96,15.4 41.12,15.56 41.12,22.23 | 41.12,22.23 41.12,25.08 39.85,26.35 v31.75,26.35 | v40.8,22.07 40.96,22.07 41.12,22.23
!HOME-1  (via drill 0.5)
  Top 0.406: M1.27 42.15,32.14 40.96,30.96 40.96,30.16 v41.12,30 | v38.58,36.51 v24.92,36.51 | ACT(DEC).C 4.44,49.36 v4.45,49.37
  Bottom 0.406: v41.12,30 41.12,33.97 v38.58,36.51 | v24.92,36.51 17.78,36.51 4.92,49.37 v4.45,49.37
!HOME-2  (via drill 0.5)
  Top 0.406: M2.27 42.62,8.49 42.23,8.1 42.23,4.76 41.91,4.45 v41.91,4.13 | ACT(RA).C v5.07,44.28 v5.08,44.29
  Bottom 0.406: v41.91,4.13 41.12,3.33 36.2,3.33 34.61,4.92 27.62,4.92 22.23,10.32 22.23,17.94 8.89,31.27 8.89,40.48 v5.08,44.29
!RST-1  (via drill 0.5)
  Top 0.406: M1.16 40.88,39.29 v39.85,40.32 | IC1.37 36.82,5.86 v36.35,5.4
  Bottom 0.406: v36.35,5.4 35.56,6.19 28.26,6.19 23.5,10.95 23.5,26.35 23.34,26.51 23.34,29.53 23.97,30.16 26.99,30.16 28.26,31.43 28.26,34.77 33.81,40.32 v39.85,40.32
!RST-2  (via drill 0.5)
  Top 0.406: M2.16 42.62,15.64 42.07,16.19 v42.07,16.99 | IC1.36 37.45,5.06 v36.67,4.29 | v22.54,25.72 v27.94,25.72
  Bottom 0.406: v36.67,4.29 36.2,4.29 34.92,5.56 27.94,5.56 22.86,10.64 22.86,25.4 v22.54,25.72 | v42.07,16.99 41.75,17.3 41.75,25.56 40.16,27.15 32.38,27.15 32.23,27.3 31.27,27.3 29.69,25.72 v27.94,25.72
+5V  (via drill 0.5)
  Top 0.406: 32.54,14.76 IC1.6 32.54,6.67 | M2.17 42.32,14.99 40.8,16.51 40.64,16.51 | M1.17 40.41,38.64 39.69,39.37 39.37,39.37 37.31,41.43 | 32.54,6.67 28.73,6.67 27.94,7.46 IC1.17 25.72,7.46 24.53,6.27 C18.1 | IC1.38 32.55,6.66 32.54,6.67
  Top 0.508: 32.92,19.27 32.44,19.27 31.91,18.73 31.91,15.4 32.54,14.76
  Top 0.61: 40.64,16.51 40.64,20.64 PROG.2 | C9.1 52.48,63.66 BLUETOOTH->.1 | v33.97,38.26 30.16,38.26 | 30.16,38.26 v27.3,38.26 | v16.99,40.64 R11.2 | R11.2 6.19,40.64 | R11.2 R14.1 | R11.2 6.25,45.72 R5.2 | C11.1 30.16,38.26
  Top 0.813: 36.35,24.92 PROG.2 40.74,25.5 R12.2 | 33.81,23.1 33.81,20.16 32.92,19.27 R20.2 | 33.81,23.1 33.81,23.81 34.92,24.92 36.35,24.92 | 33.81,23.1 C16.1 | 37.31,42.39 37.31,44.29 | 37.31,44.29 38.73,45.72 v38.73,47.31 39.37,47.95 IC3.1 | R6.2 37.31,42.39 | 37.31,42.39 37.31,41.43 34.13,38.26 v33.97,38.26 | C12.+ 35.08,44.29 37.31,44.29 | 36.35,24.92 v36.35,29.69
  Bottom 0.61: v38.73,47.31 38.73,49.53 40.16,50.96 40.16,57.94 45.72,63.5 BLUETOOTH->.1 | v27.3,38.26 24.92,40.64 v16.99,40.64
  Bottom 0.813: v33.97,38.26 33.97,34.61 36.35,32.23 v36.35,29.69
A1-1
  Top 0.406: M1.5 49.65,34.09
  Top 0.61: 49.65,34.09 49.69,34.13 50.01,34.13
  Top 1.016: 50.01,34.13 60.48,34.13 60.64,34.29 DEC.5
  Top 1.27: DEC.5 60.64,36.04 62.39,37.78 64.93,37.78 67.63,35.08 71.75,35.08 73.66,36.99 MOTOR2.8
A1-2
  Top 0.406: M2.5 50.13,10.44
  Top 0.61: 50.13,10.44 50.16,10.48 50.48,10.48
  Top 1.016: 50.48,10.48 54.29,10.48 59.05,15.24 59.05,17.14 RA.5
  Top 1.27: RA.5 60.64,20.16 62.39,21.91 64.77,21.91 67.63,19.05 70.48,19.05 71.75,20.32 71.75,20.5 73.66,22.41 MOTOR2.4
A2-1  (via drill 0.6)
  Top 0.406: M1.7 49.68,35.39
  Top 0.61: 49.68,35.39 50,35.39 50.01,35.4
  Top 1.016: 50.01,35.4 50.01,35.39 v53.02,35.39 v53.02,35.4
  Bottom 1.016: v53.02,35.4 58.9,29.53 58.9,28.73 59.85,27.78 61.12,27.78 63.18,29.84 DEC.2
  Bottom 1.27: MOTOR2.7 70.92,30.8 DEC.2
A2-2  (via drill 0.6)
  Top 0.406: M2.7 50.16,11.74
  Top 0.61: 50.16,11.74 50.48,11.74 50.48,11.75
  Top 1.016: 50.48,11.75 50.49,11.74 v53.49,11.74 v53.5,11.75
  Top 1.27: MOTOR2.3 69.04,14.92 RA.2 63.18,13.34 61.59,11.75 v57.78,11.75
  Bottom 1.016: v53.5,11.75 v57.78,11.75
AVROSC1
  Top 0.406: IC1.15 24.14,9.06 23.5,8.41 X1.P$1 23.24,8.32 22.38,7.46 C21.1
AVROSC2
  Top 0.406: C20.1 X1.P$2 23.5,11.43 25.06,9.86 IC1.14
B1-1  (via drill 0.5)
  Top 0.406: M1.10 v47.71,37.34 v47.7,37.34
  Top 1.27: MOTOR2.5 73.66,26.99 71.91,28.73 71.91,29.05 70.01,30.96 66.52,30.96 63.34,27.78 59.85,27.78 58.9,28.73 58.9,30.32 DEC.3
  Bottom 1.016: v47.7,37.34 47.74,37.31 51.12,37.31 51.91,38.1 54.45,38.1 60.48,32.07 DEC.3
B1-2  (via drill 0.5)
  Top 0.406: M2.10 v48.19,13.69 v48.18,13.68
  Bottom 1.016: v48.18,13.68 48.21,13.65 51.59,13.65 52.39,14.45 54.93,14.45 55.88,13.49 58.9,13.49
  Bottom 1.27: MOTOR2.1 72.71,12.54 70.64,14.61 65.25,14.61 62.39,11.75 60.01,11.75 58.9,12.86 58.9,13.49 58.9,14.45 RA.3
B2-1  (via drill 0.5, 0.6)
  Top 0.406: M1.8 v47.71,36.04 v47.7,36.04
  Top 1.016: v53.98,36.67 v55.88,38.58
  Top 1.27: MOTOR2.6 70.36,33.34 DEC.4
  Bottom 1.016: v47.7,36.04 v47.71,36.04 51.75,36.04 52.39,36.67 v53.98,36.67 | v55.88,38.58 63.02,38.58 64.93,36.67 64.93,35.08 DEC.4
B2-2  (via drill 0.5, 0.6)
  Top 0.406: M2.8 v48.18,12.39
  Top 1.016: v54.45,13.02 v56.36,14.92
  Bottom 1.016: v48.18,12.39 v48.19,12.38 52.23,12.38 52.86,13.02 v54.45,13.02 | v56.36,14.92 56.83,14.92 58.9,16.99 58.9,19.53 61.12,21.75 63.98,21.75 65.41,20.32 65.41,17.46
  Bottom 1.27: RA.4 65.41,17.46 72.24,17.46 MOTOR2.2
CP1-1
  Top 0.406: M1.1 48.42,31.51 48.42,30.8 48.82,30.4 C1.1
CP1-2
  Top 0.406: M2.1 48.9,7.86 48.9,7.14 49.29,6.75 C5.1
CP2-1
  Top 0.406: M1.2 47.86,32.14 47.62,31.91 47.62,30.8 47.07,30.24 C1.2
CP2-2
  Top 0.406: M2.2 48.34,8.49 48.1,8.26 48.1,7.14 47.54,6.59 C5.2
D+  (via drill 0.5)
  Top 0.279: IC2.19 1.96,14.71 v1.91,14.76
  Top 0.406: USB->.D+ 12.06,7.62 arc90 13.34,8.89 13.34,9.37 arc90 12.22,10.64 arc-90 11.27,11.75 11.27,13.49 arc90 10.05,14.71 IC2.19
  Bottom 0.279: ICSP.4 1.82,18.18 2.7,17.3 2.7,15.56 v1.91,14.76
D-  (via drill 0.5)
  Top 0.279: IC2.18 2.74,15.36 ICSP.5
  Top 0.406: v12.7,11.59 arc-90 11.91,12.38 11.91,13.49 arc90 10.2,15.36 IC2.18
  Bottom 0.406: USB->.D- 8.42,9.69 arc-90 9.53,10.79 11.91,10.79 arc90 v12.7,11.59
DIR-1  (via drill 0.5)
  Top 0.406: M1.20 40.19,36.69 39.05,35.56 29.21,35.56 v22.38,28.73 | v21.91,19.84 21.91,18.26 22.7,17.46 24.29,17.46 25.4,16.35 25.4,10.95 25.69,10.66 IC1.13
  Bottom 0.406: v21.91,19.84 22.23,20.16 22.23,24.61 21.59,25.24 21.59,26.19 22.38,26.99 v22.38,28.73
DIR-2  (via drill 0.5)
  Top 0.406: M2.20 41.46,13.04 41.12,12.7 v40.96,12.7 | IC1.9 30.14,14.31 29.05,15.4 v29.05,15.72
  Bottom 0.406: v40.96,12.7 39.85,13.81 30.64,13.81 29.05,15.4 v29.05,15.72
GND  (via drill 0.6, 2)
  Top 0.406: M1.25 45.3,33.44 46.35,32.38 v46.35,32.07 | M2.25 45.45,9.79 v46.83,8.41
  other vias: 29.37,3.49 21.11,17.62 70.48,6.35 74.77,35.24 4.6,38.73 18.73,29.69 19.05,38.42 21.11,12.54 21.11,10.32 4.45,42.7 43.97,53.66 14.92,53.82 14.92,64.29 14.92,60.96 31.91,20.32 64.77,48.74 24.61,37.94 30.64,28.42 26.83,1.11 4.45,28.26 32.07,45.4 74.93,21.27 64.45,58.42 32.54,24.92 10.95,16.51 17.14,9.53 21.11,7.94 49.05,26.04 27.62,24.29 38.1,1.11 7.78,11.11 14.92,29.53 14.92,57.15 4.29,19.37 38.73,14.92 50.32,57.31 14.29,10.64 10,11.91 5.4,8.26 13.02,6.51 14.13,12.38 12.22,15.72 14.45,7.78 13.18,13.81 19.68,15.08 10,13.49 31.59,50.16 50.32,53.82 74.93,14.45 17.62,18.89 59.05,40.64 16.19,35.24 44.13,57.31 20,33.66 30.32,7.62 33.81,3.33 66.36,27.94 33.5,7.62 36.83,55.24 46.35,43.18 4.45,33.18 38.42,51.75 59.37,22.54 25.56,46.51 72.39,48.58 55.09,55.72 45.88,12.06 45.24,8.41 45.24,15.72 46.83,15.72 44.77,32.07 45.4,35.72 44.77,39.37 46.35,39.37 18.41,23.18 15.88,21.91 39.85,6.35 39.85,9.21
  pour Top (isolate 0.406, rank 2): 43.18,66.04 77.31,66.04 77.31,0 44.45,0 44.45,40.64 43.18,41.91
  pour Top (isolate 0.254, rank 2): 0.48,0.48 44.45,0.48 44.45,46.67 43.81,47.31 43.81,50.96 44.93,52.07 53.34,52.07 59.69,58.42 59.69,64.77 58.9,65.56 0.48,65.56
  pour Bottom (isolate 0.254, rank 2): 0.48,0.48 44.45,0.48 44.45,46.67 43.81,47.31 43.81,50.96 44.93,52.07 53.34,52.07 59.69,58.42 59.69,64.77 58.9,65.56 0.48,65.56
  pour Bottom (isolate 0.406, rank 2): 43.18,66.04 77.31,66.04 77.31,0 44.45,0 44.45,40.64 43.18,41.91
ISENA-1  (via drill 0.5, 0.6)
  Top 0.406: M1.6 47.71,34.74 v47.7,34.73
  Top 1.27: R1.2 54.29,32.01 | 54.29,32.01 R2.2 | 54.29,32.01 v54.29,32.23
  Bottom 1.016: v47.7,34.73 47.74,34.77 51.75,34.77 v54.29,32.23
ISENA-2  (via drill 0.5, 0.6)
  Top 0.406: M2.6 v48.19,11.09 v48.18,11.08
  Top 1.27: R7.2 54.77,8.36 | 54.77,8.36 R8.2 | 54.77,8.36 54.77,8.89 v54.45,8.89
  Bottom 1.016: v48.18,11.08 48.21,11.11 52.23,11.11 v54.45,8.89
ISENB-1
  Top 0.406: M1.9 49.67,36.69
  Top 0.61: 50.01,36.67 49.69,36.67 49.67,36.69
  Top 1.016: 50.01,36.67 50.8,36.67 51.75,37.62 51.75,40.64
  Top 1.27: 51.75,40.64 51.7,40.64 R3.2 R4.2
ISENB-2
  Top 0.406: M2.9 50.14,13.04
  Top 0.61: 50.48,13.02 50.16,13.02 50.14,13.04
  Top 1.016: 50.48,13.02 51.28,13.02 52.23,13.97 52.23,16.99
  Top 1.27: 52.23,16.99 52.17,16.99 R9.2 R10.2
LED1
  Top 0.406: R6.1 41.59,42.39 ERR1.A
LED2
  Top 0.406: R5.1 4.07,46.51 ACT(DEC).A
LED3
  Top 0.406: ERR2.A 42.55,25.4 42.39,25.56 R12.1
LED4
  Top 0.406: R11.1 3.75,41.43 ACT(RA).A
M0-1  (via drill 0.5)
  Top 0.406: M1.24 40.92,34.09 39.85,33.02 32.7,33.02 v32.54,32.86 | IC1.42 36.34,9.86 v36.2,10
  Bottom 0.406: v36.2,10 27.3,10 25.4,11.91 25.4,26.35 31.91,32.86 v32.54,32.86
M0-2
  Top 0.406: M2.24 42.67,10.44 40.8,8.57 40.8,5.71 39.34,4.26 IC1.35
M2-1  (via drill 0.5)
  Top 0.406: M1.26 40.73,32.79 40.16,32.23 33.5,32.23 v33.18,31.91 | IC1.43 37.12,10.66 v36.83,10.95
  Bottom 0.406: v36.83,10.95 35.88,10.95 35.56,10.64 27.62,10.64 26.04,12.22 26.04,26.04 31.91,31.91 v33.18,31.91
M2-2
  Top 0.406: M2.26 42.32,9.14 41.43,8.26 41.43,5.4 39.5,3.46 IC1.34
MCLR  (via drill 0.5)
  Top 0.406: IC2.4 14.47,16.01 13.97,16.51 13.97,18.73 v12.22,20.48 | R18.1 4.37,22.68 ICSP.1
  Bottom 0.406: v12.22,20.48 10.02,22.68 ICSP.1
MISO  (via drill 0.5)
  Top 0.406: IC1.2 35.74,15.21 35.88,15.35 v35.88,15.4
  Bottom 0.406: v35.88,15.4 34.61,15.4 33.18,16.83 33.18,20.48 PROG.1
MOSI
  Top 0.406: IC1.1 36.54,14.16 38.73,16.35 39.05,16.35 39.85,17.14 39.85,18.89 PROG.4
N$1
  Top 0.406: M1.3 49.6,32.79 49.85,32.54 49.85,28.73 49.37,28.26 C3.2
N$2
  Top 0.406: IC2.9 16.56,19.26 17.3,20 17.3,21.27 18.1,22.07 20,22.07 20.8,21.27 23.42,21.27 C19.1
PWRLED
  Top 0.406: R14.2 3.91,36.36 POWER.A
RESET  (via drill 0.5)
  Top 0.406: 34.14,16.36 IC1.4 v34.13,11.59 | 34.14,16.36 PROG.5 | R20.1 32.92,17.57 34.13,16.35 34.14,16.36 | v27.15,17.78 27.15,18.1 26.12,19.13 C19.2
  Bottom 0.406: v27.15,17.78 26.67,17.3 26.67,12.54 27.94,11.27 33.81,11.27 v34.13,11.59
RX(BTH)  (via drill 0.5)
  Top 0.406: IC1.7 31.74,14.61 30.96,15.4 v30.96,16.03 | v27.3,22.07 26.35,22.07 25.24,23.18 21.75,23.18 18.89,26.04 16.51,26.04 | 16.51,26.04 12.96,26.04 R16.1 | BLUETOOTH->.4 39.37,55.88 16.51,33.02 16.51,26.04
  Bottom 0.406: v30.96,16.03 30.96,17.14 28.26,19.84 27.94,19.84 27.3,20.48 v27.3,22.07
RX(USB)
  Top 0.406: IC2.12 9.58,19.26 11.43,21.11 R16.2
SCLK  (via drill 0.5)
  Top 0.406: IC1.3 34.94,15.89 35.4,16.35 v36.99,16.35 | v27.46,19.05 24.61,21.91 21.11,21.91 18.73,24.29 v17.62,24.29 | R13.1 v11.43,30.48
  Bottom 0.406: PROG.3 33.97,18.73 33.97,17.14 34.77,16.35 v36.99,16.35 36.99,14.92 36.51,14.45 31.11,14.45 30,15.56 30,17.14 28.1,19.05 v27.46,19.05 | v17.62,24.29 v11.43,30.48
STATLED
  Top 0.406: R13.2 3.75,31.28 STATUS.A
STEP-1  (via drill 0.5)
  Top 0.406: M1.22 41.11,35.39 39.53,33.81 v31.91,33.81 | IC1.26 30.94,3.16 v30.96,3.17
  Bottom 0.406: v31.91,33.81 24.77,26.67 24.77,11.59 26.99,9.37 35.24,9.37 35.56,9.05 38.58,9.05 43.02,4.6 43.02,3.81 41.75,2.54 36.04,2.54 34.29,4.29 32.07,4.29 v30.96,3.17
STEP-2  (via drill 0.5)
  Top 0.406: M2.22 42.22,11.74 40.8,10.32 v40.48,10.32 | IC1.10 29.34,14.15 28.1,15.4 28.1,16.03 v28.89,16.83
  Bottom 0.406: v40.48,10.32 40.8,10.64 40.8,11.59 39.21,13.18 30.32,13.18 28.1,15.4 28.1,16.03 v28.89,16.83
TX(BTH)  (via drill 0.5)
  Top 0.406: IC1.5 33.34,15.39 v33.18,15.56 | R15.1 14.23,25.24 18.73,25.24 21.43,22.54 24.92,22.54 26.67,20.8 v28.26,20.8 28.26,22.38 27.62,23.02 26.35,23.02 25.56,23.81 22.07,23.81 19.05,26.83 18.1,26.83 17.3,27.62 17.3,32.54 39.85,55.09 51.12,55.09 51.59,54.61 53.02,54.61 53.66,55.24 53.66,56.52 52.32,57.85 BLUETOOTH->.3
  Bottom 0.406: v33.18,15.56 33.18,15.88 v28.26,20.8
TX(USB)
  Top 0.406: IC2.10 14.7,19.91 13.49,21.11 R15.2
USBLED
  Top 0.406: R19.1 3.43,26.2 USB.A
USBOSC1
  Top 0.406: IC2.2 18.31,14.71 18.89,14.13 X2.P$2 C15.1
USBOSC2
  Top 0.406: IC2.3 18.38,15.36 18.89,15.88 X2.P$1 C14.1
USBSTAT
  Top 0.406: IC2.16 7.29,16.66 6.99,16.97 6.99,24.13 6.99,24.29 6.99,24.34 R19.2
V+  (via drill 0.5, 0.6)
  Top 0.406: M2.4 v48.19,9.79 v48.18,9.79 | M2.11 50.11,14.34 50.16,14.29 | M1.4 v47.71,33.44 v47.7,33.44 | M1.11 49.64,37.99 49.69,37.94
  Top 0.61: 50.16,14.29 50.48,14.29 | 49.69,37.94 50.01,37.94
  Top 1.016: 50.48,14.29 50.8,14.61 v50.8,15.08 | 50.01,37.94 50.32,38.26 v50.32,38.73 | D1.C v62.71,43.81 | C4.+ 43.96,49.06 IC3.2
  Top 1.27: D1.C 61.04,43.81 C10.1 | 60.64,43.66 49.37,43.66 C4.+
  Top 1.676: 61.04,43.81 61.04,43.97 60.96,43.97 60.64,43.66
  Bottom 0.813: 59.21,24.77 52.23,17.78 50.8,17.78
  Bottom 0.965: 59.21,24.77 75.41,24.77
  Bottom 1.016: v48.18,9.79 51.65,9.79 53.82,7.62 55.09,7.62 56.83,9.37 66.67,9.37 67.94,8.1 73.66,8.1 76.36,10.79 76.36,23.81 75.41,24.77 76.36,25.72 76.36,40.01 72.55,43.81 v62.71,43.81 | v47.7,33.44 50.54,33.44 59.21,24.77
  Bottom 1.27: C8.+ 50.8,17.94 50.8,17.78 v50.8,15.08 | C4.+ 47.15,47.78 50.32,44.61 v50.32,38.73
VBUS
  Top 0.406: D2.2 9.73,9.21 USB->.VBUS
VCP-2
  Top 0.406: M2.3 50.07,9.14 50.32,8.89 50.32,5.4 49.69,4.76 C7.2
VIN
  Top 1.676: D1.A 68.47,53.04 | 68.47,53.04 J1.VIN1 | J1.VIN0 68.47,53.04
VPIC  (via drill 0.5)
  Top 0.406: 15.16,9.29 15.53,9.66 IC2.1 14.51,14.06 13.34,15.24 13.34,17.46 v11.27,19.53 | C17.1 16.03,8.41 15.16,9.29 | D2.1 14.72,9.29 15.16,9.29 | R18.2 4.57,21.18 ICSP.2
  Bottom 0.406: v11.27,19.53 9.37,21.43 1.59,21.43 1.43,21.27 ICSP.2
VUSB
  Top 0.406: IC2.17 6.53,16.01 5.87,16.67 C13.2 5.71,16.67

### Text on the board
tNames: Thomas Carpenter (2012) | 12v (4A Max) | A1 | A2 | B2 | S2 | B1 | A1 | A2 | B2 | B1 | AstroEQ | Controller | V3.0-SMD

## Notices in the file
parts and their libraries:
SparkFun: Licensing: CC v3.0 Share-Alike You are welcome to use this library for commercial purposes.
